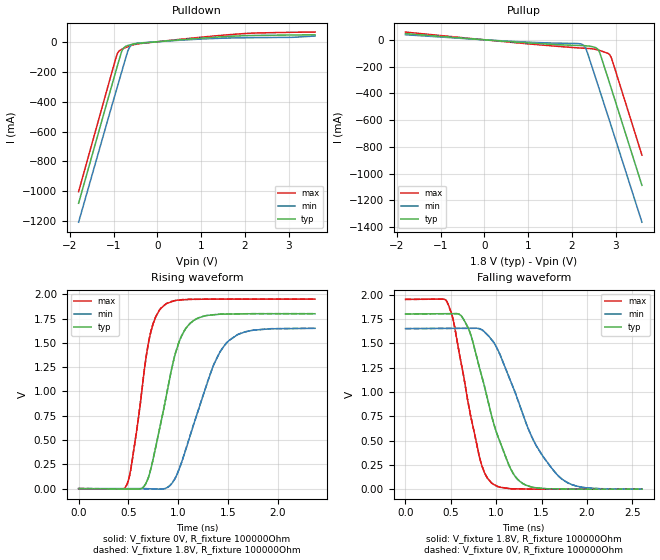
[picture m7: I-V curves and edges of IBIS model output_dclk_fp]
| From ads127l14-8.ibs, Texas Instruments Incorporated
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|   output_dclk_fp Model
[Model]   output_dclk_fp
Model_type   Output
Polarity   Non-Inverting
Vmeas = 0.9
Vref = 0
Cref = 2pF
Rref = 100000
|   typ   min   max
C_comp   0.469pF   0.517pF   0.451pF
[Voltage Range]   1.8   1.65   1.95
[Temperature Range]   27   125   -40
[Pullup Reference]   1.8   1.65   1.95
[Pulldown Reference]   0   0   0
[Power Clamp Reference]   1.8   1.65   1.95
[GND Clamp Reference]   0   0   0
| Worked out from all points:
|   slope of the pulldown table from 0 to 0.27 V, typ, clamps not added: 39.9 ohm
|   slope of the pullup table from 0 to 0.27 V, typ, clamps not added: 41.3 ohm
|   falling waveform, V_fixture 1.8V, R_fixture 100000Ohm: 20-80 % time 330ps typ, 452ps min, 239ps max; typ from 1.8 V to 0.001 V
|   rising waveform, V_fixture 0V, R_fixture 100000Ohm: 20-80 % time 227ps typ, 324ps min, 161ps max; typ from 0 V to 1.8 V
|   rising waveform, V_fixture 1.8V, R_fixture 100000Ohm: 20-80 % time 227ps typ, 325ps min, 161ps max; typ from 0.001 V to 1.8 V
|   falling waveform, V_fixture 0V, R_fixture 100000Ohm: 20-80 % time 330ps typ, 452ps min, 239ps max; typ from 1.8 V to 0 V
[Pulldown]
|   Voltage   I(typ)   I(min)   I(max)
-1.8V     -1.08A     -1.206A    -1.002A
-919.8mV  -167.2mA   -305.8mA   -83.63mA
-876.6mV  -123.2mA   -262.2mA   -62.69mA
-822.6mV  -70.29mA   -207.7mA   -52.02mA
-774mV    -42.2mA    -158.8mA   -45.36mA
-671.4mV  -24.61mA   -59.09mA   -32.47mA
-639mV    -21.83mA   -38.19mA   -28.81mA
-590.4mV  -18.32mA   -21.03mA   -23.92mA
-444.6mV  -11.5mA    -9.358mA   -14.43mA
235.8mV   5.927mA    4.679mA    7.417mA
1.834V    38.58mA    25.73mA    51.49mA
3.6V      46.23mA    38.16mA    64.43mA
[Pullup]
|   Voltage   I(typ)   I(min)   I(max)
-1.8V     45.88mA    37.72mA    57.48mA
765mV     -18.04mA   -13.93mA   -23.34mA
2.131V    -42.16mA   -28.04mA   -60.12mA
2.261V    -43.57mA   -39.85mA   -62.81mA
2.309V    -44.48mA   -60.52mA   -63.75mA
2.358V    -45.88mA   -99.81mA   -64.72mA
2.542V    -58.22mA   -283.8mA   -71.74mA
2.612V    -79.58mA   -354.4mA   -77.4mA
2.639V    -98.68mA   -381.5mA   -79.98mA
2.822V    -283.9mA   -567.1mA   -101.4mA
2.887V    -350.4mA   -633mA     -124.4mA
3.6V      -1.087A    -1.363A    -861.4mA
[Ramp]
R_load = 100000
|   typ   min   max
dV/dt_r   1.07956/2.25599e-10   0.989492/3.2244e-10   1.16963/1.60295e-10
dV/dt_f   1.07958/3.29747e-10   0.989512/4.50999e-10   1.16963/2.38486e-10
[Falling Waveform]
V_fixture = 1.8V
V_fixture_min = 1.65V
V_fixture_max = 1.95V
R_fixture = 100000Ohm
C_fixture = 0F
|   Time   V(typ)   V(min)   V(max)
0s        1.8V       1.65V      1.95V
457.8ps   1.803V     1.652V     1.926V
532.8ps   1.804V     1.653V     1.711V
696.7ps   1.646V     1.653V     860mV
839.7ps   1.165V     1.639V     248.7mV
947.2ps   761.8mV    1.539V     65.75mV
1.232ns   105.5mV    933.5mV    3.291mV
1.418ns   17mV       488.8mV    626.9uV
1.669ns   2.972mV    151.4mV    626.9uV
2.606ns   734.6uV    809.6uV    626.9uV
[Rising Waveform]
V_fixture = 0V
V_fixture_min = 0V
V_fixture_max = 0V
R_fixture = 100000Ohm
C_fixture = 0F
|   Time   V(typ)   V(min)   V(max)
0s        1.317nV    13.69nV    11.96nV
486.3ps   -3.634mV   187.9uV    42.96mV
525.4ps   -3.927mV   203uV      203.2mV
710.8ps   143.7mV    -906.3uV   1.545V
883.2ps   962.8mV    7.978mV    1.903V
971.8ps   1.388V     109.4mV    1.935V
1.08ns    1.652V     410.3mV    1.945V
1.347ns   1.787V     1.247V     1.949V
1.482ns   1.796V     1.493V     1.949V
2.376ns   1.799V     1.649V     1.949V
[Rising Waveform]
V_fixture = 1.8V
V_fixture_min = 1.65V
V_fixture_max = 1.95V
R_fixture = 100000Ohm
C_fixture = 0F
|   Time   V(typ)   V(min)   V(max)
0s        706.9uV    813.3uV    614.2uV
478.4ps   -2.857mV   -2.173mV   26.61mV
536.4ps   -3.29mV    -2.535mV   273.7mV
675.2ps   51.61mV    -3.401mV   1.332V
752.8ps   323.3mV    -3.886mV   1.709V
851.3ps   798.9mV    -1.84mV    1.881V
1.069ns   1.635V     378.7mV    1.945V
1.347ns   1.788V     1.248V     1.95V
1.497ns   1.796V     1.511V     1.95V
2.376ns   1.8V       1.65V      1.95V
[Falling Waveform]
|Gnd
V_fixture = 0V
V_fixture_min = 0V
V_fixture_max = 0V
R_fixture = 100000Ohm
C_fixture = 0F
|   Time   V(typ)   V(min)   V(max)
0s        1.799V     1.649V     1.949V
457.8ps   1.802V     1.651V     1.925V
532.8ps   1.803V     1.652V     1.71V
696.7ps   1.645V     1.653V     859mV
839.7ps   1.164V     1.638V     247.8mV
947.2ps   760.6mV    1.538V     65.07mV
1.232ns   104.6mV    932mV      2.674mV
1.418ns   16.26mV    487.2mV    12.73uV
1.669ns   2.259mV    150.1mV    12.73uV
2.606ns   27.65uV    -3.75uV    12.73uV
